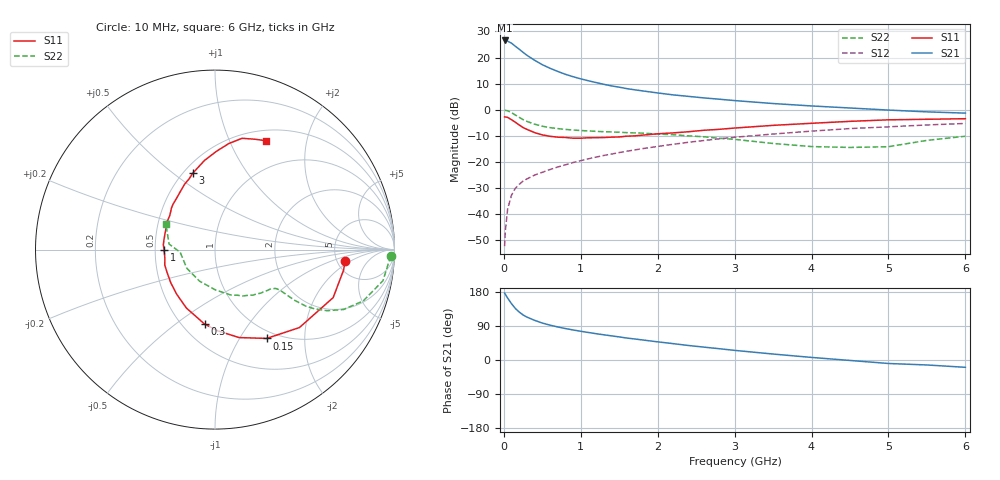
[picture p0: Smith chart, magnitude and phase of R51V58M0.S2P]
! SIEMENS Small Signal Semiconductors
! BFR183
! Si NPN RF Bipolar Junction Transistor in SOT23
! VCE = 1.5 V  IC = 8 mA
! Common Emitter S-Parameters:  May  1996
# GHz  S  MA  R  50
!  f  S11  S21  S12  S22
! GHz  MAG  ANG  MAG  ANG  MAG  ANG  MAG  ANG
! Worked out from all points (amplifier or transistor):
!   36 points, 10 MHz to 6 GHz, reference 50 ohm
!   highest |S21| = 26.6 dB at 10 MHz (marker M1)
!   |S21| within 3 dB of that: start of sweep to 183.9 MHz
!   unconditionally stable (mu >= 1): 800.2 MHz to 2.566 GHz
!   at 250 MHz: K = 0.57, MSG = 24.7 dB, |S12| = -27.4 dB
!   at 1.4 GHz: K = 1.07, MAG = 11.5 dB, |S12| = -17.0 dB
!   at 6 GHz: K = 0.91, MSG = 2.0 dB, |S12| = -5.3 dB
!   S11 on the Smith chart (normalised r, x): 10 MHz: 5.91, -1.56; 150 MHz: 0.89, -1.32; 300 MHz: 0.64, -0.64; 1 GHz: 0.56, -0.00; 3 GHz: 0.56, +0.59; 6 GHz: 0.63, +1.38
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0.01  0.7272 -4.9  21.28 176.7  0.0024 83.7  0.9821 -2.1
0.02  0.7255 -9.0  20.99 173.1  0.0048 84.8  0.9705 -4.2
0.05  0.7107 -22.1  20.61 163.2  0.0126 79.7  0.9517 -10.5
0.1  0.6403 -42.7  18.85 148.5  0.0229 71.5  0.8741 -19.1
0.15  0.5726 -59.8  16.45 135.9  0.031 65.4  0.7899 -25.0
0.2  0.5081 -74.7  14.45 126.5  0.0369 62.3  0.7113 -28.6
0.25  0.4538 -87.7  12.6 118.9  0.0426 60.0  0.6441 -30.8
0.3  0.4188 -98.0  11.06 113.2  0.0468 59.5  0.5956 -31.9
0.4  0.3625 -116.1  8.868 104.7  0.0555 58.7  0.5271 -32.5
0.5  0.3279 -130.5  7.291 97.5  0.0628 59.7  0.4806 -32.3
0.6  0.3083 -142.9  6.228 92.0  0.0709 60.7  0.452 -32.1
0.7  0.2964 -153.6  5.422 87.3  0.0793 61.5  0.4333 -32.1
0.8  0.2929 -162.7  4.771 83.0  0.0873 61.5  0.4175 -32.2
1  0.2832 -179.3  3.901 75.8  0.1051 62.3  0.3978 -32.9
1.1  0.2891 174.7  3.581 72.6  0.114 62.4  0.3905 -34.0
1.6  0.3101 148.5  2.531 57.9  0.1593 60.6  0.3621 -39.7
2.2  0.3579 126.6  1.922 43.2  0.2162 56.0  0.3307 -50.1
3  0.4436 106.2  1.494 25.4  0.2951 47.6  0.2693 -70.4
3.5  0.4996 96.8  1.311 15.7  0.3407 41.4  0.2244 -89.5
4.5  0.5965 82.5  1.076 -1.2  0.4337 28.7  0.1883 -146.5
5.5  0.6539 70.1  0.907 -13.1  0.5089 16.7  0.2573 173.2
6  0.6703 64.9  0.858 -19.3  0.5436 8.8  0.3087 152.6
